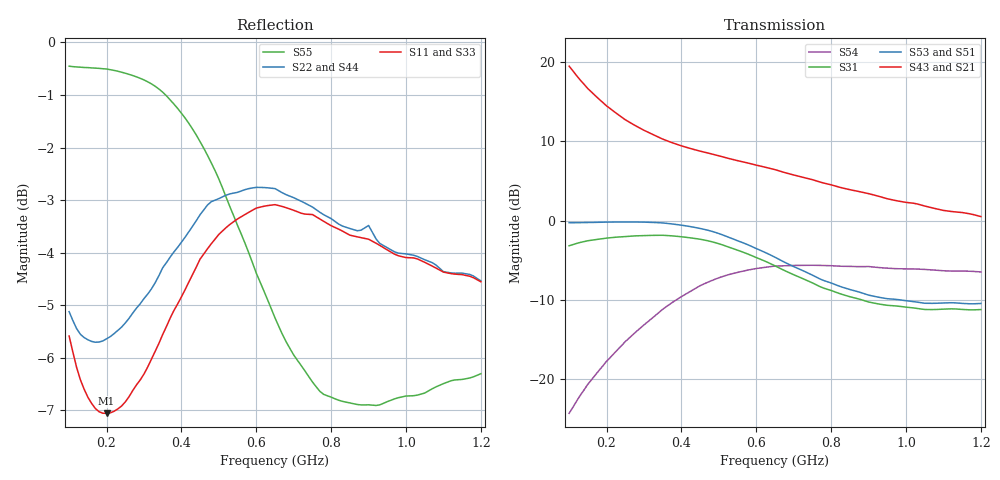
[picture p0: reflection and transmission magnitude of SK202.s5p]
!  POLYFET RF DEVICES
!  S PARAMETERS FOR
!  SK202 (Each Side)
!  VDS=28, IDQ=400MA
! S2A2Die, AP pkg,
! Date: Thu Sep 24 14:52:01 1998
!AWR Design Environment (2053) Wed Feb 04 15:23:10 2004
!freq-unit  param-type  data-format  keyword  impedance-ohms
# MHz  S  MA  R  50
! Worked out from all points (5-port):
!   111 points, 100 MHz to 1.2 GHz, reference 50 ohm
!   strongest paths, dB at 100 MHz, 370 MHz, 650 MHz, 930 MHz, 1.2 GHz:
!     S43: 19.4, 9.9, 6.4, 3.0, 0.5
!     S21: 19.4, 9.9, 6.4, 3.0, 0.5
!     S53: -0.3, -0.4, -4.6, -9.7, -10.4
!     S51: -0.3, -0.4, -4.6, -9.7, -10.4
!     S31: -3.2, -1.9, -5.7, -10.5, -11.2
!     S54: -24.3, -10.5, -5.7, -5.9, -6.5
!   lowest |S11| = -7.1 dB at 200 MHz (marker M1), VSWR 2.60, Z = 51.9 - j50.4 ohm
!   |S11| at or under -10 dB: nowhere
